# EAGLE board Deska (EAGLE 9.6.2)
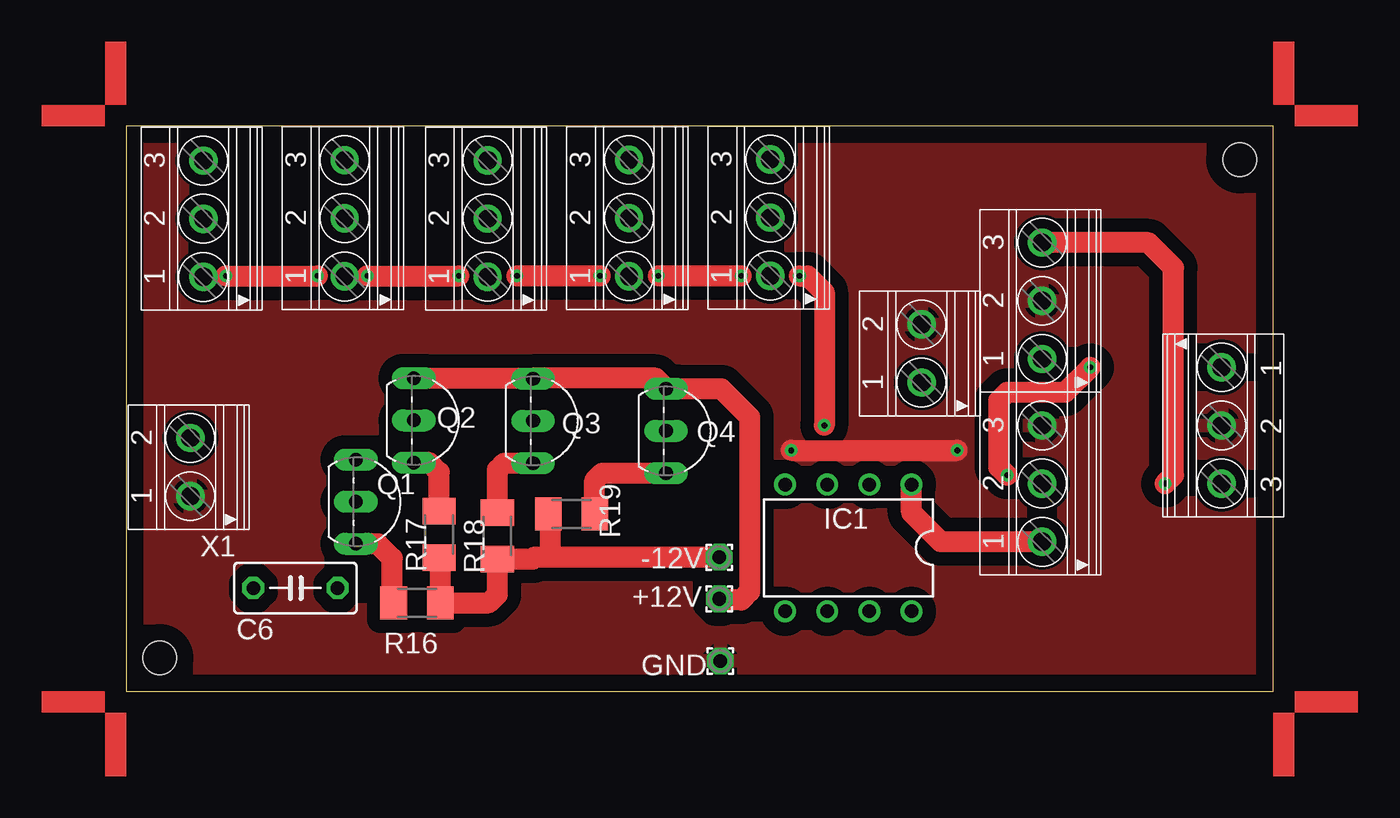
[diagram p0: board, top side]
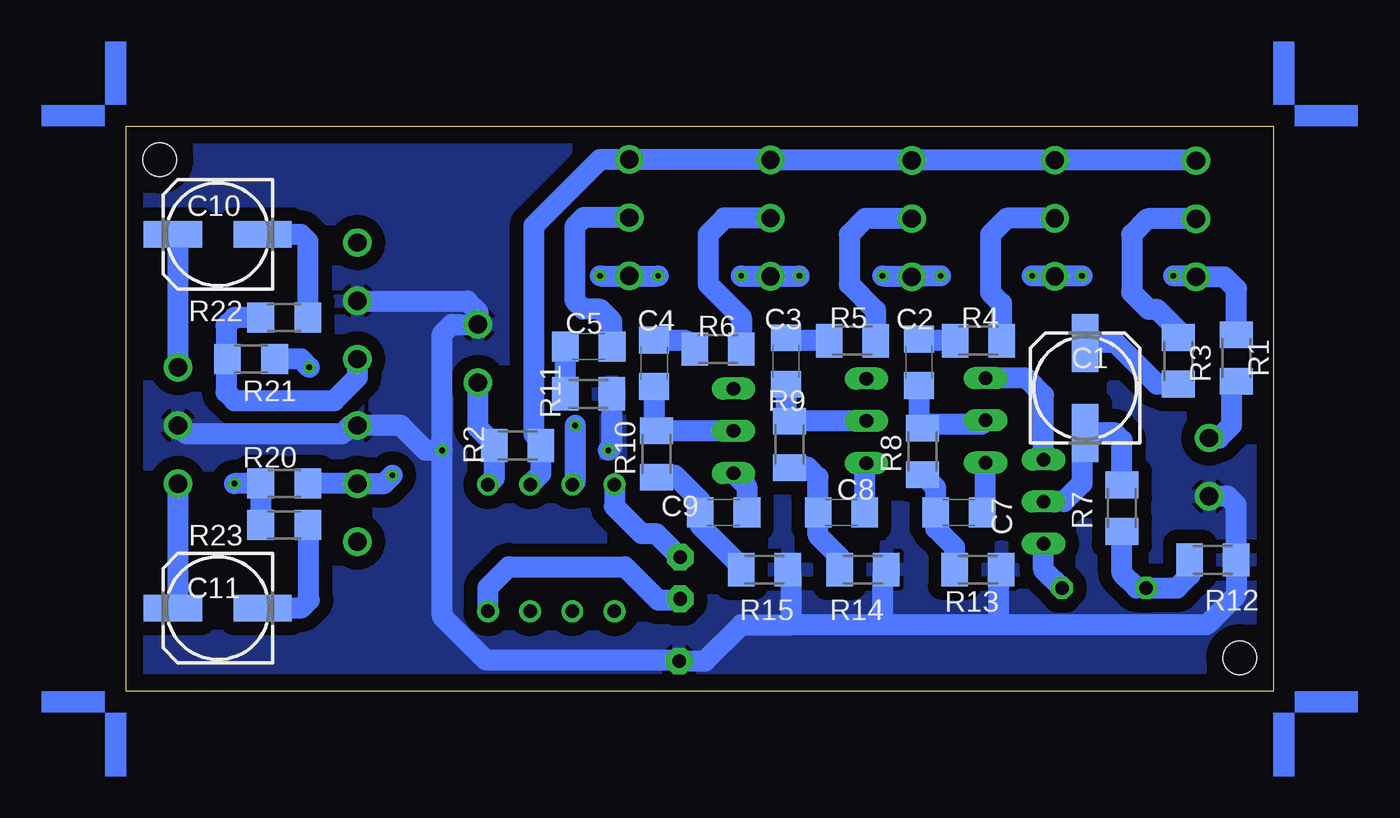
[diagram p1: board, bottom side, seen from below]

Size 69 x 34 mm. Coordinates in mm from the lower left corner, seen from the top.
Outline: 0,0 69,0 69,34 0,34 0,0
Copper layers (1*16): Top 0.035mm / dielectric 1.5mm / Bottom 0.035mm
Design rules "default": minimum track width 6mil, minimum drill 0.35mm, track to track 6mil, track to pad 6mil, pad to pad 6mil, via to via 6mil, smd to smd 6mil, copper to edge 40mil, drill to drill 6mil, minimum pad ring 10mil, minimum via ring 8mil, stop-mask expansion 4mil, vias tented up to drill 0mil, thermal gap 10mil
Holes 2 mm at 67,32 2,2

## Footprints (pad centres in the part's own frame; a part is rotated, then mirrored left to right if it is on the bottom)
1,6/0,8 = drill 0.813 pad 1.6 octagon: 1 0,0
153CLV-0605 = smd 3.5 x 1.6: + 2.7,0; - -2.7,0
C1206 = smd 1.6 x 1.8: 1 -1.4,0; 2 1.4,0
C050-030X075 = drill 0.813 octagon: 1 -2.54,0; 2 2.54,0
DIL08 = drill 0.813 pad 1.27: 1 -3.81,-3.81; 2 -1.27,-3.81; 3 1.27,-3.81; 4 3.81,-3.81; 5 3.81,3.81; 6 1.27,3.81; 7 -1.27,3.81; 8 -3.81,3.81
TO92-EBC = drill 0.813 long: B 0,-1.27; C -2.54,-1.27; E 2.54,-1.27
M1206 = smd 1.6 x 2: 1 -1.4,0; 2 1.4,0
R1206 = smd 1.6 x 1.803: 1 -1.422,0; 2 1.422,0
1751248 = drill 1.1 pad 1.7: 1 -1.75,-0.1; 2 1.75,-0.1
1751251 = drill 1.1 pad 1.7: 1 -3.5,-0.1; 2 0,-0.1; 3 3.5,-0.1

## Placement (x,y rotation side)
+12V  [1,6/0,8]  35.68,5.56 0 top
-12V  [1,6/0,8]  35.68,8.06 90 top
C1  [153CLV-0605]  11.31,18.25 90 bottom
C2  [C1206]  21.32,19.8 270 bottom
C3  [C1206]  29.32,19.88 270 bottom
C4  [C1206]  37.24,19.74 270 bottom
C5  [C1206]  41.18,20.74 180 bottom
C6  [C050-030X075]  10.17,6.21 0 top
C7  [C1206]  18.9,10.76 0 bottom
C8  [C1206]  25.98,10.76 0 bottom
C9  [C1206]  33.06,10.76 0 bottom
C10  [153CLV-0605]  63.5,27.5 180 bottom
C11  [153CLV-0605]  63.5,5 180 bottom
GND  [1,6/0,8]  35.74,1.82 90 top
IC1  NE5532N  [DIL08]  43.44,8.63 180 top
Q1  BC549C  [TO92-EBC]  15.08,11.41 270 top
Q2  BC549C  [TO92-EBC]  18.58,16.3 270 top
Q3  BC549C  [TO92-EBC]  25.74,16.28 270 top
Q4  BC549C  [TO92-EBC]  33.74,15.67 270 top
R1  [M1206]  2.21,20.05 90 bottom
R2  [M1206]  45.47,14.79 180 bottom
R3  [M1206]  5.71,19.89 90 bottom
R4  [M1206]  17.74,21.1 0 bottom
R5  [M1206]  25.32,21.1 0 bottom
R6  [M1206]  33.4,20.6 0 bottom
R7  [M1206]  9.1,11.02 90 bottom
R8  [M1206]  21.1,14.44 90 bottom
R9  [M1206]  29.1,14.86 90 bottom
R10  [M1206]  37.1,14.28 90 bottom
R11  [M1206]  41.2,17.9 180 bottom
R12  [M1206]  3.62,7.9 180 bottom
R13  [M1206]  17.76,7.32 180 bottom
R14  [M1206]  24.68,7.32 180 bottom
R15  [M1206]  30.6,7.32 180 bottom
R16  [M1206]  17.48,5.32 180 top
R17  [M1206]  18.82,9.44 90 top
R18  [M1206]  22.32,9.36 90 top
R19  [M1206]  26.78,10.68 0 top
R20  [R1206]  59.5,12.5 180 bottom
R21  [R1206]  61.5,20 180 bottom
R22  [R1206]  59.5,22.5 0 bottom
R23  [R1206]  59.5,10 0 bottom
U$1  [ANGLE-SW1-16]  69,34 0 top
U$2  [ANGLE-SW1-16]  0,34 90 top
U$3  [ANGLE-SW1-16]  0,0 180 top
U$4  [ANGLE-SW1-16]  69,0 270 top
X1  [1751248]  3.75,13.49 90 top
X2  [1751248]  47.75,20.33 90 top
X3  [1751251]  4.53,28.44 90 top
X4  [1751251]  13.03,28.47 90 top
X5  [1751251]  21.64,28.45 90 top
X6  [1751251]  30.14,28.48 90 top
X7  [1751251]  38.64,28.51 90 top
X8  [1751251]  55,12.5 90 top
X9  [1751251]  55,23.5 90 top
X10  [1751251]  66,16 270 top

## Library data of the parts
+12V -12V GND = wirepad
C1-C11 = rcl; SPICEPREFIX: C
IC1 = linear
Q1-Q4 = transistor-npn
R1-R23 = rcl; SPICEPREFIX: R
U$1-U$4 = marks
X1-X10 = con-phoenix-350; OC_FARNELL: unknown; OC_NEWARK: unknown

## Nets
GND: GND.1 R11.1 R12.1 R13.1 R14.1 R15.1 X1.1 X2.2 X8.3 X9.2 X10.2
N$1: IC1.1 R2.2 X2.1 X8.1
N$2: R1.1 X1.2
N$3: IC1.3 R1.2 X3.1 X4.1 X5.1 X6.1 X7.1
N$4: IC1.2 R2.1 X3.3 X4.3 X5.3 X6.3 X7.3
N$5: R3.2 X3.2
N$6: R4.2 X4.2
N$7: R5.2 X5.2
N$8: R6.2 X6.2
N$9: C1.+ R3.1
N$10: C2.1 R4.1
N$11: C3.1 R5.1
N$12: C4.1 R6.1
N$13: C5.1 X7.2
N$14: C5.2 R11.2
N$15: C1.- Q1.B R7.2
N$16: C2.2 Q2.B R8.2
N$17: C3.2 Q3.B R9.2
N$18: C4.2 Q4.B R10.2
N$19: +12V.1 IC1.8 Q1.C Q2.C Q3.C Q4.C
N$20: C6.1 R7.1 R12.2
N$21: C7.1 R8.1 R13.2
N$22: C8.1 R9.1 R14.2
N$23: C9.1 R10.1 R15.2
N$24: C9.2 Q4.E R19.2
N$25: C8.2 Q3.E R18.2
N$26: C7.2 Q2.E R17.2
N$27: C6.2 Q1.E R16.2
N$28: -12V.1 IC1.4 R16.1 R17.1 R18.1 R19.1
N$29: R20.1 R21.1 X8.2
N$30: R21.2 R22.1 X9.1
N$31: R20.2 R23.1 X9.3
N$32: C11.- R23.2
N$33: C10.- R22.2
N$34: C10.+ X10.1
N$35: C11.+ X10.3

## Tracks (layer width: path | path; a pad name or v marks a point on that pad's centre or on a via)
GND  (via drill 0.35)
  Top 1.27: v40,14.5 v50,14.5
  Bottom 1.27: X1.1 2.74,11.74 2.22,11.22 R12.1 2.22,5.78 4,4 16.5,4 | 16.5,4 16.5,7.18 R13.1 | 16.5,4 23.5,4 | R14.1 23.5,7.1 23.5,4 | 23.5,4 29,4 | R15.1 29,7.12 29,4 | 29,4 32,4 34.18,1.82 GND.1 35.79,1.87 47.35,1.87 50,4.52 v50,14.5 | v50,14.5 50,21.5 49.42,22.08 X2.2 47.85,22.85 48.5,23.5 X9.2 | R11.1 39.8,14.7 v40,14.5 | v50,14.5 51,14.5 52.5,16 X8.3 55.5,16 56,15.5 65.4,15.5 X10.2
  pour Top (isolate 0.813): 0,0 69,0 69,34 0,34
  pour Bottom (isolate 0.813): 0,0 69,0 69,34 0,34
N$1
  Top 1.27: X8.1 49,9 47.25,10.75 IC1.1
  Bottom 1.27: IC1.1 46.87,12.82 R2.2 46.87,14.87 47.85,15.85 X2.1
N$2
  Bottom 1.27: R1.1 2.5,18.36 2.5,16 3.26,15.24 X1.2
N$3  (via drill 0.35)
  Top 1.27: v37,25 v32,25 | v28.5,25 v23.5,25 | v14.5,25 v20,25 | v6,25 v11.5,25 | v40.5,25 41,25 42,24 v42,16
  Bottom 1.27: v40.5,25 X7.1 v37,25 | v32,25 31.98,24.98 X6.1 28.52,24.98 v28.5,25 | v23.5,25 21.79,25 | 21.79,25 X5.1 | v14.5,25 13.16,25 X4.1 13.1,25 v11.5,25 | v20,25 21.79,25 | v6,25 4.69,25 X3.1 2.94,24.94 2.21,24.21 R1.2 | v42,16 42,12.61 IC1.3
N$4
  Bottom 1.27: X3.3 4.66,31.97 X4.3 21.72,31.97 X5.3 21.77,31.98 X6.3 30.27,32.01 X7.3 40.49,32.01 44.5,28 44.5,15.5 44.07,15.07 R2.1 44.07,13.08 IC1.2
N$5
  Bottom 1.27: X3.2 7.56,28.44 8.5,27.5 8.5,24 7.5,23 7,23 5.71,21.71 R3.2
N$6
  Bottom 1.27: X4.2 16.03,28.47 17,27.5 17,24 16.34,23.34 R4.2
N$7
  Bottom 1.27: X5.2 24.55,28.45 25.5,27.5 25.5,24.5 23.92,22.92 R5.2
N$8
  Bottom 1.27: X6.2 33.02,28.48 34,27.5 34,24.5 32,22.5 R6.2
N$9
  Bottom 1.27: C1.+ 11.27,20.99 9.49,20.99 6.99,18.49 R3.1
N$10
  Bottom 1.27: R4.1 21.22,21.1 C2.1
N$11
  Bottom 1.27: C3.1 29.14,21.1 R5.1
N$12
  Bottom 1.27: C4.1 37.2,21.1 35.3,21.1 R6.1
N$13
  Bottom 1.27: X7.2 41.49,28.51 42,28 42,23.5 41.5,23 40.5,23 39.78,22.28 C5.1
N$14
  Bottom 1.27: C5.2 42.6,20.72 R11.2
N$15
  Bottom 1.27: R7.2 9.1,15.1 9.55,15.55 C1.- 11.5,15.36 11.5,12.5 12.59,11.41 Q1.B
N$16
  Bottom 1.27: C2.2 21.32,16.06 | 21.32,16.06 R8.2 | Q2.B 17.55,16.06 21.32,16.06
N$17
  Bottom 1.27: 29.5,18.3 C3.2 29.32,16.48 29.12,16.28 | 29.12,16.28 R9.2 | Q3.B 29.12,16.28
N$18
  Bottom 1.27: Q4.B R10.2 37.24,15.82 C4.2
N$19
  Top 1.27: Q2.C 24.45,18.84 | 24.45,18.84 Q3.C | 24.45,18.84 31.84,18.84 Q4.C 35.79,18.21 37.5,16.5 37.5,6 37,5.5 35.74,5.5 +12V.1
  Bottom 1.27: Q1.C 13.81,17.81 14.84,18.84 Q2.C | IC1.8 47.25,6.25 46,7.5 39,7.5 37,5.5 35.74,5.5 +12V.1
N$20
  Bottom 1.27: R7.1 9.1,7.1 8.21,6.21 C6.1 5.79,6.21 5,7 5,7.88 R12.2
N$21
  Bottom 1.27: R8.1 20.3,12.24 C7.1 20.3,9.8 19.16,8.66 R13.2
N$22
  Bottom 1.27: R9.1 29.06,13.5 28,13.5 27.38,12.88 C8.1 27.38,9.38 26.08,8.08 R14.2
N$23
  Bottom 1.27: R10.1 36.98,13 36,13 34.46,11.46 C9.1 34.46,9.96 32,7.5 R15.2
N$24
  Top 1.27: R19.2 28.18,12.68 28.63,13.13 Q4.E
  Bottom 1.27: Q4.E 31.66,12.32 C9.2
N$25
  Top 1.27: R18.2 22.32,13.32 22.74,13.74 Q3.E
  Bottom 1.27: Q3.E 24.58,13.63 C8.2
N$26
  Top 1.27: R17.2 18.82,13.18 18.24,13.76 Q2.E
  Bottom 1.27: C7.2 17.31,10.95 Q2.E
N$27
  Top 1.27: R16.2 16,5.4 16,8 15.13,8.87 Q1.E
  Bottom 1.27: C6.2 13.81,7.31 Q1.E
N$28
  Top 1.27: R17.1 18.88,7.98 R16.1 21.82,5.32 22.32,5.82 R18.1 24.46,7.96 24.56,8.06 25.5,8.06 | -12V.1 25.5,8.06 | R19.1 25.5,10.56 25.5,8.06
  Bottom 1.27: IC1.4 39.63,11.13 38,9.5 37.12,9.5 -12V.1
N$29  (via drill 0.35)
  Top 1.27: v53,13 52.5,13.5 52.5,17.5 53,18 56.5,18 v58,19.5
  Bottom 1.27: R20.1 X8.2 53.5,12.5 v53,13 | v58,19.5 58.5,20 R21.1
N$30
  Bottom 1.27: R22.1 62.5,22.5 63,22 63,20.08 R21.2 63,19.92 63,18 62.5,17.5 56.5,17.5 55.1,18.9 X9.1
N$31  (via drill 0.35)
  Top 1.27: v62.5,12.5 63,13 63,25.5 61.5,27 X9.3
  Bottom 1.27: R23.1 R20.2 v62.5,12.5
N$32
  Bottom 1.27: R23.2 58.08,5.58 58,5.5 58.5,5 C11.- 60.92,5.12
N$33
  Bottom 1.27: R22.2 58.08,27.08 58.5,27.5 C10.- 60.92,27.38
N$34
  Bottom 1.27: C10.+ 65.9,27.2 X10.1
N$35
  Bottom 1.27: X10.3 65.9,5.3 C11.+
